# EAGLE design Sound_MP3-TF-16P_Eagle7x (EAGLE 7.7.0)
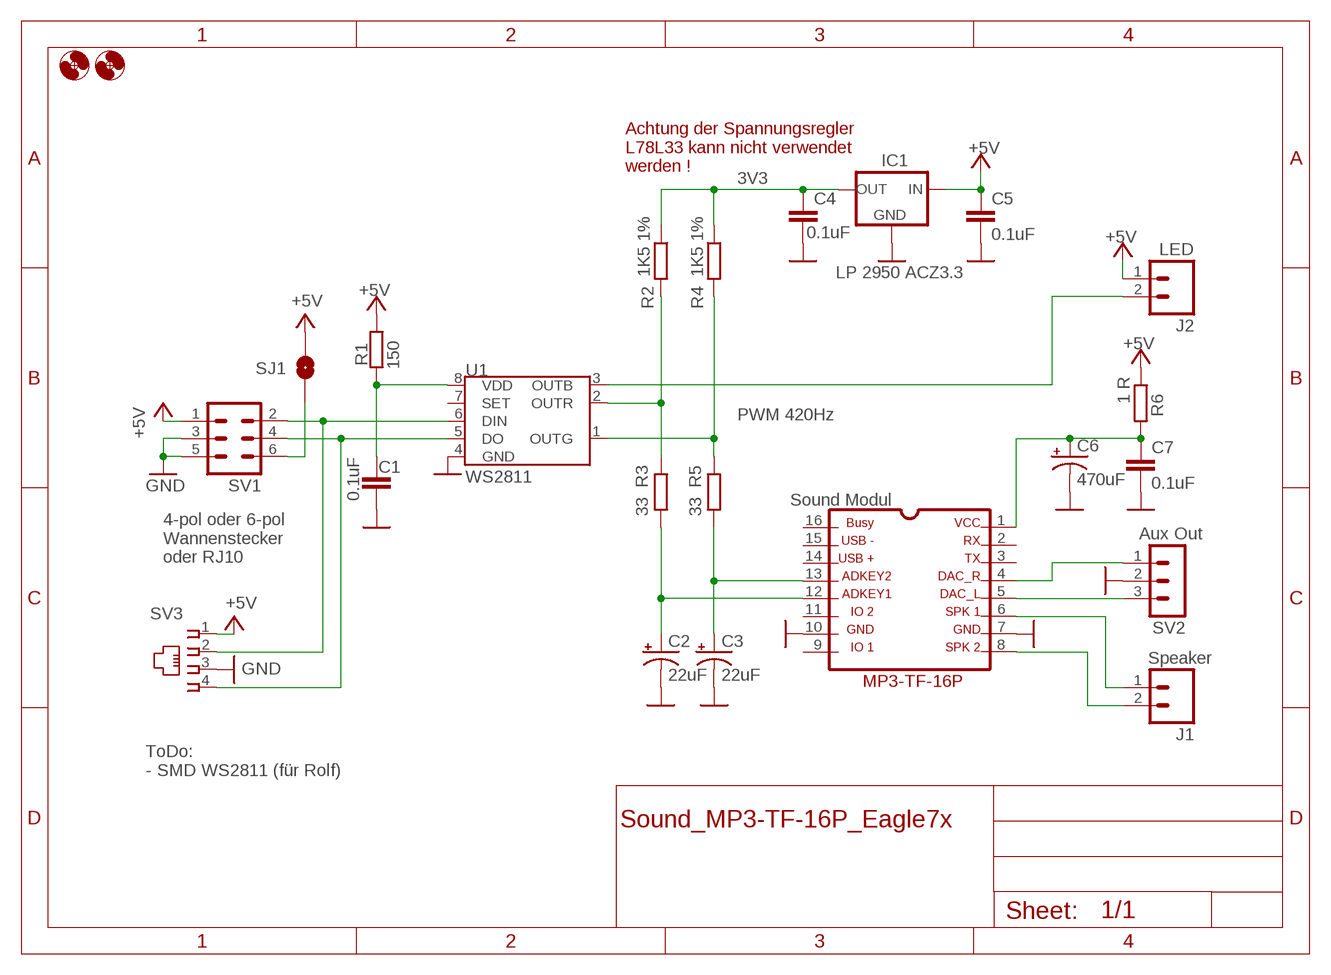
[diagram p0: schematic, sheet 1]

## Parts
C1  0.1uF  0.1UF-50V-20%(PTH)KIT-EZ  [CAP-PTH-SMALL-KIT]
C2  22uF  CAPACITORS_22UF  [CAPACITOR_CPOL-RADIAL-22UF]
C3  22uF  CAPACITORS_22UF  [CAPACITOR_CPOL-RADIAL-22UF]
C4  0.1uF  0.1UF-50V-20%(PTH)KIT-EZ  [CAP-PTH-SMALL-KIT]
C5  0.1uF  0.1UF-50V-20%(PTH)KIT-EZ  [CAP-PTH-SMALL-KIT]
C6  470uF  SPARKFUN-CAPACITORS_100UF-25V-20%(PTH)  [SPARKFUN-CAPACITORS_CPOL-RADIAL-100UF-25V]
C7  0.1uF  0.1UF-50V-20%(PTH)KIT-EZ  [CAP-PTH-SMALL-KIT]
H1  MOUNT-HOLE3.0  [3,0]
H3  MOUNT-HOLE3.0  [3,0]
IC1  LP 2950 ACZ3.3  78LXX  [78LXX]
J1  Speaker  M02PTH  [1X02]
J2  LED  M02PTH  [1X02]
MOD1  Sound Modul  MP3-TF-16P_MP3-TF-16P  [MP3-TF-16P_MP3-TF-16P]
R1  150  RCL_R-EU_0204/5  [RCL_0204/5]
R2  1K5 1%  RCL_R-EU_0204/5  [RCL_0204/5]
R3  33  RCL_R-EU_0204/5  [RCL_0204/5]
R4  1K5 1%  RCL_R-EU_0204/5  [RCL_0204/5]
R5  33  RCL_R-EU_0204/5  [RCL_0204/5]
R6  1 R  RCL_R-EU_0204/5  [RCL_0204/5]
SJ1  Pin6 = 5V  SOLDERJUMPERNO  [SJ_2S-NO]
SV1  ML6  [ML6]
SV2  Aux Out  MA03-1  [MA03-1]
SV3  RJ10RJ10_WO_OVERLAP  [RJ10_NO_OVERLAP_BORDER]
U1  WS2811  S3PO_MODUL_WS2811_SOUND_MP3-TF-16P_WS2811_AND_ATTINY_WS2811-ICTINY45-20-DIP  [S3PO_MODUL_WS2811_SOUND_MP3-TF-16P_WS2811_AND_ATTINY_WS2811_DIP08]

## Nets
3V3: C4.1 IC1.OUT R2.1 R4.1
+5V: C5.1 IC1.IN J2.1 R1.2 R6.1 SJ1.1 SV1.1 SV3.1
+5V1: SJ1.2 SV1.6
G1: R4.2 R5.1 U1.1(OUTG)
GND: C1.2 C2.2(-) C3.2(-) C4.2 C5.2 C6.2(-) C7.2 IC1.GND MOD1.7 MOD1.10 SV1.3 SV1.5 SV2.2 SV3.3 U1.4(GND)
N$1: MOD1.5 SV2.3
N$2: MOD1.4 SV2.1
N$3: SV1.2 SV3.2 U1.6(DIN)
N$4: SV1.4 SV3.4 U1.5(DO)
N$5: J1.1 MOD1.6
N$6: J1.2 MOD1.8
N$7: C2.1(+) MOD1.12 R3.2
N$8: C3.1(+) MOD1.13 R5.2
N$9: C6.1(+) C7.1 MOD1.1 R6.2
N$10: J2.2 U1.3(OUTB)
PWR1: C1.1 R1.1 U1.8(VDD)
R1: R2.2 R3.1 U1.2(OUTR)
Unconnected: MOD1.2 MOD1.3 MOD1.9 MOD1.11 MOD1.14 MOD1.15 MOD1.16 U1.7(SET)

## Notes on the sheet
- Achtung der Spannungsregler
  L78L33 kann nicht verwendet
  werden !
- PWM 420Hz
- 4-pol oder 6-pol 
  Wannenstecker
  oder RJ10
- ToDo:
  - SMD WS2811 (für Rolf)

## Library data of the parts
C1 C4 C5 C7 = SparkFun-Capacitors:0.1UF-50V-20%(PTH): CAP-08370; PROD_ID: CAP-08370
C2 C3 = Sound_MP3-TF-16P_WS2811_and_ATTiny:CAPACITORS_22UF: CAP-08439; PROD_ID: CAP-08439
C6 = Sound_MP3-TF-16P_and_WS2811:SPARKFUN-CAPACITORS_100UF-25V-20%(PTH): CAP-08439; PROD_ID: CAP-08439
H1 H3 = holes:MOUNT-HOLE: MOUNTING HOLE with drill center marker
IC1 = v-reg-3:78LXX: VOLTAGE REGULATOR
J1 J2 = SparkFun-Connectors:M02: Standard 2-pin 0.1" header. Use with
MOD1 = Sound_MP3-TF-16P_WS2811_and_ATTiny:MP3-TF-16P_MP3-TF-16P: MP3-TF-16P http://www.electronicoscaldas.com/datasheet/DFR0299-DFPlayer-Mini-Manual.pdf; OC_FARNELL: unknown; OC_NEWARK: unknown
R1-R6 = Sound_MP3-TF-16P_and_WS2811:RCL_R-EU_: RESISTOR, European symbol; SPICEPREFIX: R
SJ1 = SparkFun-Retired:SOLDERJUMPER: Solder Jumper
SV1 = con-harting-ml:ML6: HARTING; OC_FARNELL: unknown; OC_NEWARK: unknown
SV2 = con-lstb:MA03-1: PIN HEADER
SV3 = RJ10:RJ10: RJ10 Connector "C:\Dat\Märklin\Schaltpläne\Allgemein\RJ10_Stecker_Layout.docx" ...
U1 = S3PO_Modul_WS2811:S3PO_MODUL_WS2811_SOUND_MP3-TF-16P_WS2811_AND_ATTINY_WS2811-IC: Die Pin nummern im Dokument https://cdn-shop.adafruit.com/datasheets/WS2811.pdf für R und G sind vertauscht ;-(; PROD_ID: IC-09439; VALUE: TINY45-20-DIP

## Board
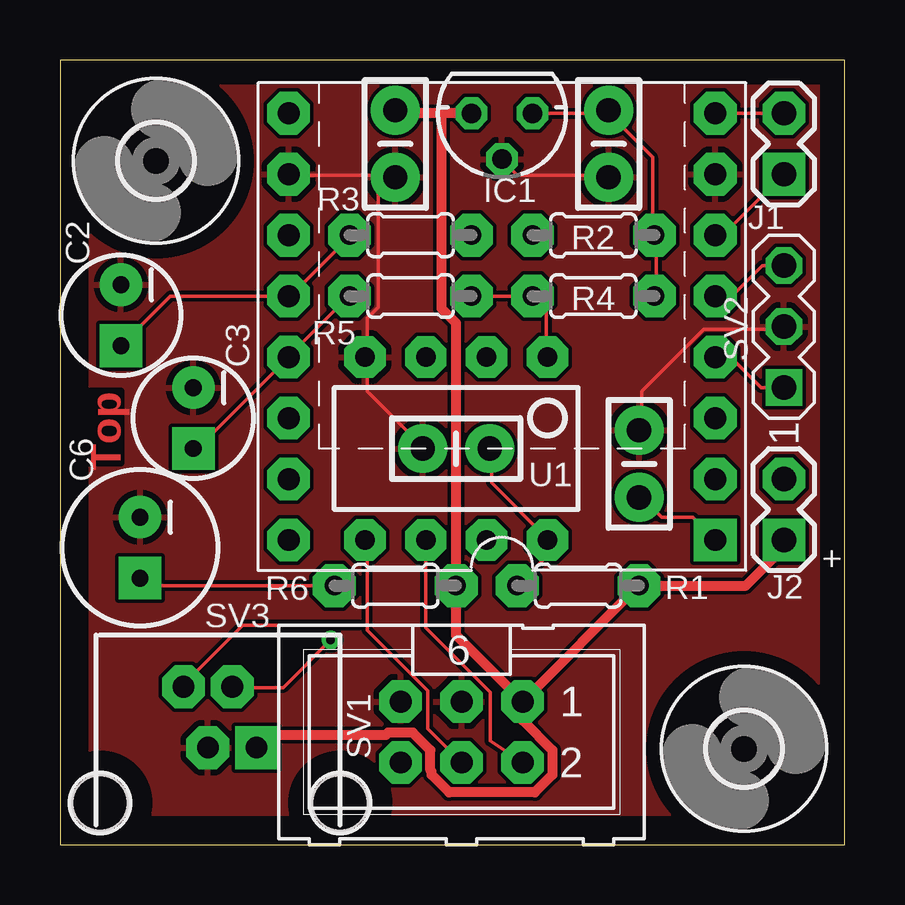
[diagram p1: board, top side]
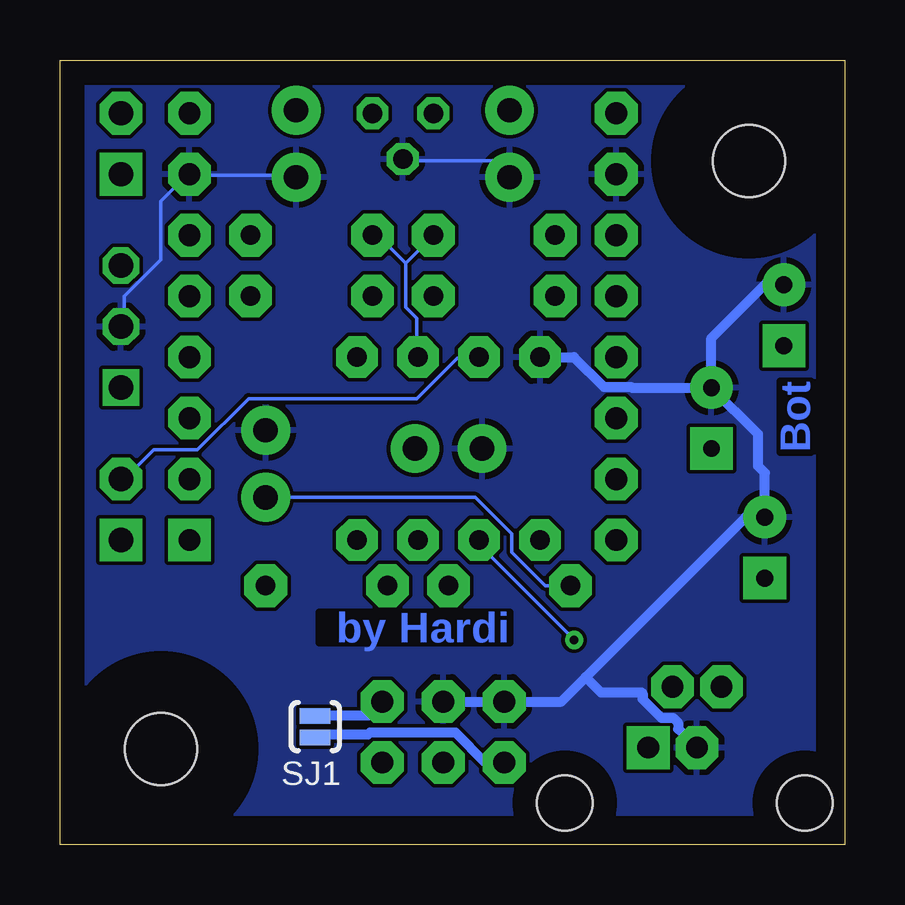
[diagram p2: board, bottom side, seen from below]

Size 32.7 x 32.7 mm. Coordinates in mm from the lower left corner, seen from the top.
Outline: 0,0 32.7,0 32.7,32.7 0,32.7 0,0
Copper layers (1*16): Top 0.035mm / dielectric 1.5mm / Bottom 0.035mm
Design rules "default": minimum track width 6mil, minimum drill 0.35mm, track to track 6mil, track to pad 6mil, pad to pad 6mil, via to via 6mil, smd to smd 6mil, copper to edge 40mil, drill to drill 6mil, minimum pad ring 10mil, minimum via ring 8mil, stop-mask expansion 4mil, vias tented up to drill 0mil, thermal gap 10mil

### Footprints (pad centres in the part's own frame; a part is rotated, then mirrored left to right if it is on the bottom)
CAP-PTH-SMALL-KIT = drill 1.016 pad 2.032: 1 -1.397,0; 2 1.397,0
CAPACITOR_CPOL-RADIAL-22UF = drill 0.7 pad 1.778 square: 1 1.27,0 | drill 0.7 pad 1.778: 2 -1.27,0
SPARKFUN-CAPACITORS_CPOL-RADIAL-100UF-25V = drill 0.7 pad 1.778 square: 1 1.27,0 | drill 0.7 pad 1.778: 2 -1.27,0
3,0 = hole 3: 0,0
78LXX = drill 0.813 octagon: GND 0,1.905; IN 1.27,0; OUT -1.27,0
1X02 = drill 1.016 pad 1.778 square: 1 0,0 | drill 1.016 pad 1.778 octagon: 2 2.54,0
MP3-TF-16P_MP3-TF-16P = drill 0.914 pad 1.778 square: 1 -8.89,16.51 | drill 0.914 pad 1.778 octagon: 2 -8.89,13.97; 3 -8.89,11.43; 4 -8.89,8.89; 5 -8.89,6.35; 6 -8.89,3.81; 7 -8.89,1.27; 8 -8.89,-1.27; 9 8.89,-1.27; 10 8.89,1.27; 11 8.89,3.81; 12 8.89,6.35; 13 8.89,8.89; 14 8.89,11.43; 15 8.89,13.97; 16 8.89,16.51
RCL_0204/5 = drill 0.813 pad 1.778 octagon: 1 -2.54,0; 2 2.54,0
SJ_2S-NO = smd 0.635 x 1.27: 1 -0.45,0; 2 0.45,0
ML6 = drill 0.914 pad 1.778 octagon: 1 -2.54,-1.27; 2 -2.54,1.27; 3 0,-1.27; 4 0,1.27; 5 2.54,-1.27; 6 2.54,1.27
MA03-1 = drill 1.016 pad 1.524 square: 1 -3.81,0 | drill 1.016 pad 1.524 octagon: 2 -1.27,0; 3 1.27,0
RJ10_NO_OVERLAP_BORDER = drill 0.9 pad 1.778 square: 1 -1.524,-2.3 | drill 0.9 pad 1.778 octagon: 2 -0.508,-4.84; 3 0.508,-2.3; 4 1.524,-4.84 | hole 2.3: 5,0; -5,0
S3PO_MODUL_WS2811_SOUND_MP3-TF-16P_WS2811_AND_ATTINY_WS2811_DIP08 = drill 0.813 pad 1.727 octagon: 1 -3.81,-3.81; 2 -1.27,-3.81; 3 1.27,-3.81; 4 3.81,-3.81; 5 3.81,3.81; 6 1.27,3.81; 7 -1.27,3.81; 8 -3.81,3.81

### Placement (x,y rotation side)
C1  16.51,16.51 180 top
C2  2.54,22.07 270 top
C3  5.56,17.78 270 top
C4  22.86,29.21 270 top
C5  13.97,29.21 270 top
C6  3.33,12.38 270 top
C7  24.13,15.88 90 top
H1  4,28.5 0 top
H3  28.5,4 0 top
IC1  18.41,30.48 180 top
J1  30.16,27.94 90 top
J2  30.16,12.7 90 top
MOD1  18.41,29.21 180 top
R1  21.59,10.79 0 top
R2  22.23,25.4 180 top
R3  14.61,25.4 180 top
R4  22.23,22.86 180 top
R5  14.61,22.86 180 top
R6  13.97,10.79 180 top
SJ1  22.07,4.92 270 bottom
SV1  16.73,4.7 180 top
SV2  30.16,22.86 90 top
SV3  6.67,1.75 180 top
U1  16.51,16.51 180 top

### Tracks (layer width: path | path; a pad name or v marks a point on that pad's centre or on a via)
3V3
  Top 0.152: R4.1 24.84,22.86 24.84,25.3 R2.1 24.69,25.45 24.69,28.65 22.86,30.48 | 22.86,30.48 C4.1 | IC1.OUT 22.86,30.48
+5V
  Top 0.152: 11.43,4.57 14.63,4.57 15.39,3.81 15.39,3.1
  Top 0.406: SV1.1 24.1,10.79 R1.2 28.57,10.79 30.16,12.38 J2.1 | SV1.1 16.51,8.73 R6.1 16.51,21.73 15.9,22.34 15.9,30.45 15.88,30.48 | IC1.IN 15.88,30.48 | 15.88,30.48 14.1,30.48 C5.1 | SV1.1 19.27,5.19 20.52,3.94 20.52,2.91 19.79,2.18 16.22,2.18 15.49,2.91 15.49,3.05 15.44,3.1 15.44,3.94 14.71,4.67 13.68,4.67 13.57,4.57 11.43,4.57 8.72,4.57 SV3.1
  Bottom 0.406: SJ1.1 22.04,5.4 19.84,5.4 SV1.1
+5V1
  Bottom 0.406: SV1.6 14.97,3.43 16.22,4.67 19.79,4.67 19.86,4.6 21.93,4.6 SJ1.2
G1
  Top 0.152: U1.1 20.27,20.42 20.27,22.4 19.81,22.86 R4.2 R5.1
GND
  Top 0.152: C7.2 24.23,17.37 24.23,18.9 26.82,21.49 30.02,21.49 SV2.2 | C1.2 15.09,16.61 12.8,18.9 12.8,20.27 U1.4 12.8,20.42 12.8,21.95 13.26,22.4 13.26,27.89 | 13.26,27.89 13.87,27.89 C5.2 13.26,27.89 | 13.26,27.89 9.6,27.89 MOD1.10 9.45,27.89 | C4.2 22.86,27.89 19.05,27.89 18.44,28.5 IC1.GND
  Bottom 0.152: SV2.2 30.02,21.64 30.02,22.86 28.5,24.38 28.5,26.82 27.43,27.89 MOD1.7 27.28,27.89 22.86,27.89 C4.2 | IC1.GND 18.29,28.5 14.63,28.5 14.02,27.89 C5.2
  Bottom 0.406: SV1.3 SV1.5 11.81,5.97 10.79,6.99 | 10.79,6.99 4.13,13.65 C6.2 3.33,15.5 3.61,15.78 3.61,17.11 C3.2 | C3.2 5.56,21.11 3.33,23.34 C2.2 | 10.79,6.99 10.16,6.35 8.46,6.35 8.42,6.31 8.42,6.07 7.64,5.29 7.16,5.29 6.95,5.08 6.95,4.83 SV3.3 | U1.4 11.29,20.32 10.04,19.07 8.91,19.07 8.89,19.05 C3.2
  pour Top: 1.27,1.27 31.75,1.27 31.75,31.75 3.81,31.75 1.27,29.21 1.27,27.94
  pour Bottom: 1.27,1.27 30.48,1.27 31.75,2.54 31.75,31.75 1.27,31.75
N$1
  Top 0.152: MOD1.5 27.99,22.86 29.26,24.13 SV2.3
N$2
  Top 0.152: SV2.1 29.21,19.05 27.94,20.32 MOD1.4
N$3  (via drill 0.35)
  Top 0.152: SV1.2 17.92,4.33 17.92,6.36 15.24,9.04 U1.6 | v11.28,8.53 9.3,6.55 7.32,6.55 SV3.2
  Bottom 0.152: v11.28,8.53 15.24,12.5 U1.6
N$4
  Top 0.152: 12.8,9.14 12.8,12.65 U1.5 | SV1.4 15.32,4.84 15.32,6.43 12.8,8.94 12.8,9.14 | 12.8,9.14 7.62,9.14 5.18,6.71 SV3.4
N$5
  Top 0.152: J1.1 27.62,25.4 MOD1.6
N$6
  Top 0.152: J1.2 MOD1.8
N$7
  Top 0.152: R3.2 12.04,25.3 9.6,22.86 MOD1.12 4.6,22.86 C2.1
N$8
  Top 0.152: R5.2 12.04,22.86 9.6,20.42 MOD1.13 5.71,16.51 C3.1
N$9
  Top 0.152: C7.1 24.23,14.48 25.07,13.64 26.36,13.64 MOD1.1 | R6.2 3.65,10.79 C6.1
  Bottom 0.152: C7.1 15.39,14.48 13.87,12.95 13.87,12.19 12.47,10.79 R6.2
N$10
  Bottom 0.152: U1.3 15.24,20.27 16.15,20.27 17.83,18.59 24.84,18.59 26.98,16.46 28.8,16.46 30.02,15.24 J2.2
PWR1
  Top 0.152: C1.1 17.98,16.46 17.98,15.09 20.27,12.8 U1.8 20.32,12.06 R1.1
R1
  Bottom 0.152: 18.29,24.23 18.29,22.4 17.83,21.95 17.83,20.42 U1.2 | 18.29,24.23 17.22,25.3 R3.1 | 18.29,24.23 19.36,25.3 19.66,25.3 R2.2

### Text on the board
Top: Top
Bottom: Bot | by Hardi
tNames: +
tDocu: MP3-TF-16P | 30.10.19 | Sound Modul | V 1.0 | by Hardi
bDocu: MP3-TF-16P / Sound Modul | V 1.0 | by Hardi

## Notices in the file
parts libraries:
SparkFun-Capacitors: Licensing: Creative Commons ShareAlike 4.0 International - https://creativecommons.org/licenses/by-sa/4.0
